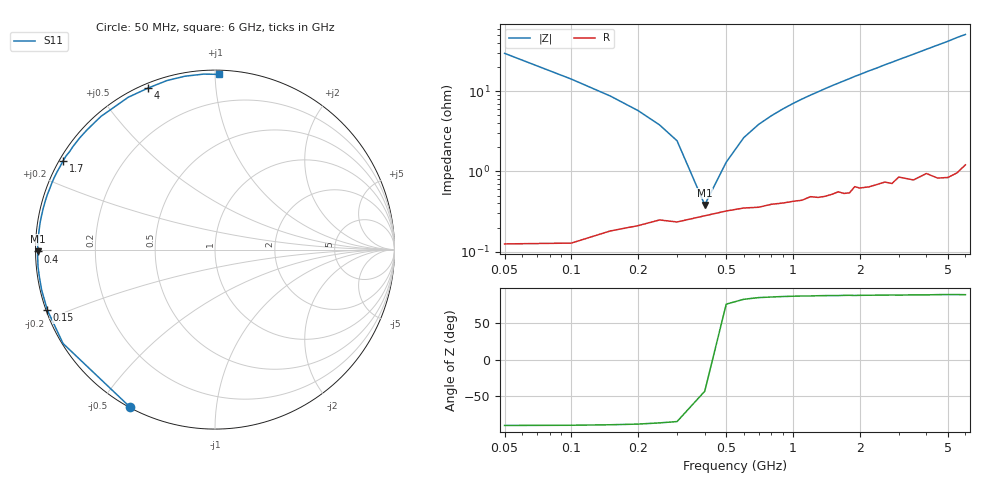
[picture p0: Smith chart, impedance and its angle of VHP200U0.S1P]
! Infineon Technologies  Discrete & RF Semiconductors
! BB 814
! Si Tuning Diode in SOT23
! VR = 0.2 V
! S-Parameters:  July  1999
# GHz  S  MA  R  50
!  f  S11
! GHz  MAG  ANG
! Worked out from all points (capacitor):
!   34 points, 50 MHz to 6 GHz, reference 50 ohm
!   read as one part to ground: C = 106 pF near 50 MHz
!   lowest |Z| = 383 mohm at 400 MHz (marker M1)
!   series resonance near 417.1 MHz, so ESL is about 1.4 nH
!   S11 on the Smith chart (normalised r, x): 50 MHz: 0.00, -0.59; 150 MHz: 0.00, -0.17; 400 MHz: 0.01, -0.01; 1.7 GHz: 0.01, +0.27; 4 GHz: 0.02, +0.67; 6 GHz: 0.02, +1.02
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0.05  0.9963 -118.5
0.1  0.9953 -148.3
0.15  0.993 -160.2
0.2  0.9917 -166.9
0.25  0.9902 -171.3
0.3  0.9907 -174.5
0.4  0.9889 -179.4
0.5  0.9872 177.1
0.6  0.9861 174.0
0.7  0.9859 171.2
0.8  0.9847 168.7
1.1  0.983 161.8
1.4  0.9814 155.6
1.6  0.9792 151.7
1.7  0.9804 149.8
1.9  0.9766 145.9
2  0.9778 144.2
2.2  0.9775 140.5
2.4  0.9764 137.2
2.6  0.9754 133.6
2.8  0.9769 130.5
3  0.973 127.2
3.5  0.9768 119.7
4  0.9742 112.5
4.5  0.9791 105.9
5  0.9805 99.9
5.5  0.9797 93.7
6  0.9767 88.7
